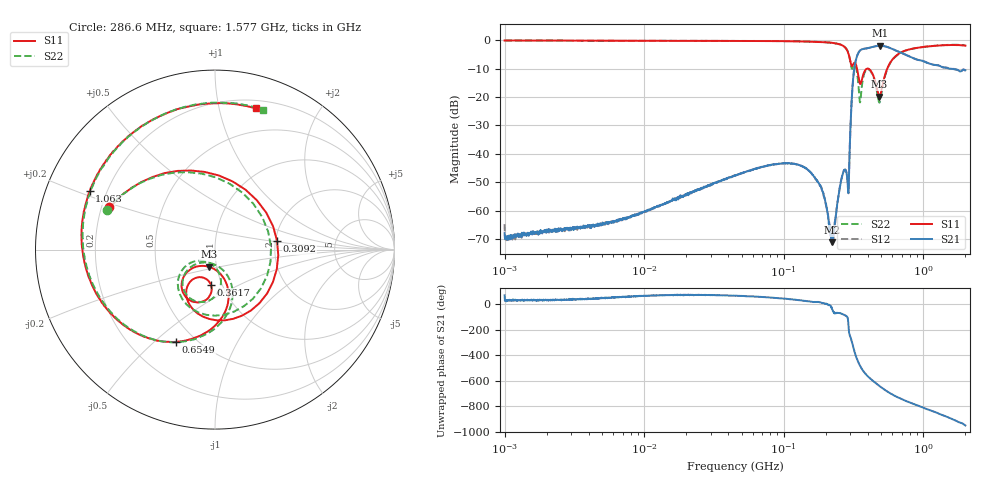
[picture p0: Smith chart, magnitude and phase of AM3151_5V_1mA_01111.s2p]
! Date/Time: Fri Jun 26 10:36:57 2020
! Network Analyzer:  Rev:
! Sweep from 1000000.0 to 2000000000.0, 1601 Points ! Power Supply: 0 V, 0 A
# HZ S DB R 50
!freq MagS11 AngS11 MagS21 AngS21 MagS12 AngS12 MagS22 AngS22
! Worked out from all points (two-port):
!   1601 points, 1 MHz to 2 GHz, reference 50 ohm
!   highest |S21| = -1.99 dB at 490.2 MHz (marker M1); lowest = -71.0 dB at 222.8 MHz (marker M2)
!   |S21| within 3 dB of the highest: 338.7 MHz to 733 MHz (394.3 MHz wide, 73.6 % of centre)
!   lowest |S11| = -19.8 dB at 483.2 MHz (marker M3), VSWR 1.23, Z = 45.8 - j8.84 ohm
!   |S11| at or under -10 dB: 334.6 MHz to 551.4 MHz (216.8 MHz wide, 48.9 % of centre)
!   |S22| runs from -22.0 to -0.1 dB; largest |S21 - S12| = 0.0082
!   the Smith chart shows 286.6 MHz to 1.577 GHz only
!   S11 on the Smith chart (normalised r, x): 286.6 MHz: 0.23, +0.18; 309.2 MHz: 2.04, +0.23; 361.7 MHz: 0.89, -0.36; 654.9 MHz: 0.40, -0.59; 1.063 GHz: 0.14, +0.22; 1.577 GHz: 0.27, +1.29
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1000000  -0.15 -0.9  -67.82 71.2  -64.69 38.4  -0.15 -0.9
3555161  -0.22 -2.0  -65.73 43.2  -65.95 41.2  -0.21 -2.0
1.263916e7  -0.28 -5.9  -58.38 70.4  -58.19 72.1  -0.27 -5.8
4.493426e7  -0.32 -19.9  -47.59 67.1  -47.39 68.1  -0.31 -19.8
1.589914e8  -0.58 -72.9  -46.97 20.4  -46.97 20.6  -0.58 -72.7
1.895438e8  -0.74 -89.5  -53.27 11.1  -53.02 11.4  -0.72 -89.3
2.227702e8  -0.98 -111.2  -71.00 -40.9  -72.40 -39.8  -1.01 -111.1
2.605798e8  -1.80 -147.9  -48.14 -74.0  -48.14 -73.4  -1.76 -147.5
2.865518e8  -3.97 158.2  -49.83 -104.6  -50.01 -104.4  -3.85 159.9
3.091819e8  -9.14 8.1  -17.95 56.6  -17.96 56.7  -10.10 2.9
3.28878e8  -8.67 -105.4  -6.90 -46.7  -6.92 -46.5  -9.59 -123.0
3.448783e8  -13.61 -126.9  -4.21 -102.6  -4.19 -102.6  -17.65 -150.2
3.616573e8  -14.14 -96.9  -3.28 -145.0  -3.28 -145.0  -16.54 -78.9
4.07264e8  -10.14 -121.1  -2.75 147.4  -2.76 147.4  -10.36 -118.5
4.832253e8  -19.85 -110.1  -2.01 80.5  -1.99 80.4  -21.95 -108.9
4.901608e8  -19.52 -95.8  -1.99 75.3  -1.99 75.3  -21.46 -89.7
5.652395e8  -8.86 -81.9  -2.60 28.8  -2.61 28.7  -8.98 -78.0
6.54923e8  -5.07 -112.8  -3.97 -8.9  -3.95 -9.1  -5.14 -111.4
8.464476e8  -2.96 -162.9  -6.36 -61.6  -6.35 -61.5  -3.02 -163.8
1.063239e9  -2.27 155.1  -8.00 -102.6  -7.95 -102.6  -2.29 152.9
1.577145e9  -1.74 73.9  -10.10 -175.6  -10.19 -175.8  -1.69 71.0
2e9  -1.97 14.0  -10.61 129.8  -10.75 129.0  -1.87 12.8
